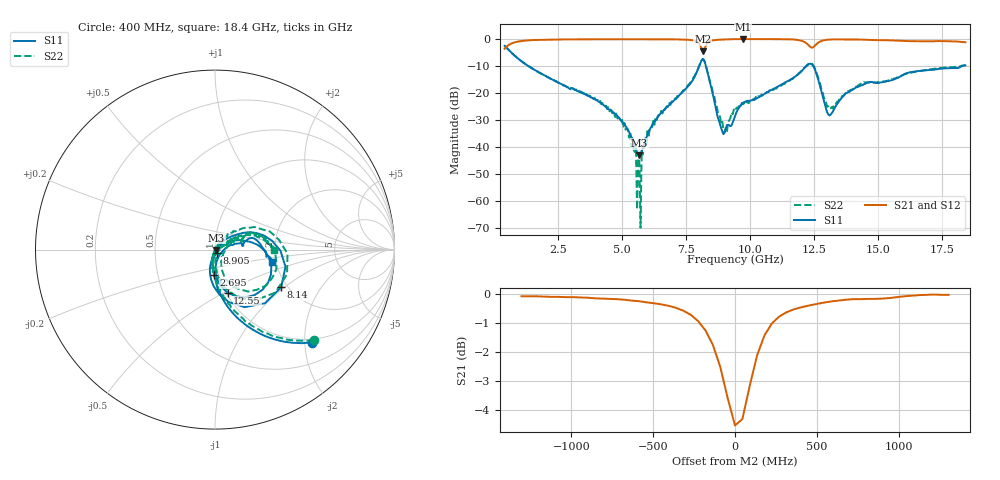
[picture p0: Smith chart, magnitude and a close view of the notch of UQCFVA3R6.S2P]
!  Part Number  UQCFVA3R6  Mounting Orientation: Horizontal
!  Description: Ultra Low ESR Microwave capacitors
!  Application: Coupling, Bypass, Tuning, DC Block
!  Filters, Matching
# GHZ S DB R 50
! Freq  |S11|  S11 Ph  |S21|  S21 Ph  |S12|  S12 Ph  |S22|  S22 Ph
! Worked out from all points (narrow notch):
!   401 points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, 400 MHz to 18.4 GHz, reference 50 ohm
!   highest |S21| = -0.01 dB at 9.715 GHz (marker M1); lowest = -4.5 dB at 8.14 GHz (marker M2)
!   notch at M2: 4.4 dB deep, 225 MHz wide at half that depth
!   lowest |S11| = -43.2 dB at 5.665 GHz (marker M3), VSWR 1.01, Z = 50.6 - j0.26 ohm
!   |S11| at or under -10 dB: 1.323 GHz to 8 GHz (6.676 GHz wide, 143 % of centre); 8.264 GHz to 12.2 GHz (3.932 GHz wide, 38.4 % of centre); 12.46 GHz to 18.29 GHz (5.837 GHz wide, 38 % of centre)
!   |S22| runs from -70.0 to -2.5 dB; largest |S21 - S12| = 0.0053
!   S11 on the Smith chart (normalised r, x): 400 MHz: 0.92, -2.15; 2.695 GHz: 0.95, -0.27; 8.14 GHz: 1.85, -0.95; 8.905 GHz: 1.02, -0.03; 12.55 GHz: 1.02, -0.52; 18.4 GHz: 1.89, -0.30
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0.4  -2.53 -43.9  -3.59 46.6  -3.60 46.6  -2.54 -42.6
1.12  -8.66 -74.2  -0.66 16.8  -0.67 16.8  -8.72 -71.6
2.695  -17.04 -91.6  -0.15 -3.1  -0.16 -3.1  -17.30 -90.5
3.415  -20.02 -96.5  -0.10 -9.1  -0.11 -9.0  -19.69 -95.4
5.08  -31.68 -94.4  -0.06 -19.7  -0.07 -19.6  -31.12 -106.3
5.44  -38.57 -77.2  -0.04 -21.9  -0.05 -21.9  -41.08 -74.8
5.665  -43.20 -21.8  -0.04 -23.3  -0.04 -23.3  -45.68 35.6
5.845  -39.20 24.0  -0.04 -24.5  -0.04 -24.5  -40.58 27.6
6.43  -28.40 45.5  -0.07 -28.4  -0.07 -28.3  -28.12 60.0
7.87  -13.01 25.6  -0.73 -44.4  -0.72 -44.2  -12.78 32.1
8.14  -7.44 -29.7  -4.55 -39.4  -4.55 -39.3  -7.45 -18.8
8.41  -15.55 -97.7  -0.79 -26.3  -0.77 -26.2  -15.39 -80.7
8.905  -34.40 -58.2  -0.19 -35.2  -0.17 -35.1  -30.76 -57.1
9.4  -28.58 31.0  -0.04 -39.4  -0.02 -39.4  -26.75 26.3
9.715  -23.69 26.1  -0.01 -41.7  -0.01 -41.7  -24.22 27.9
11.875  -13.01 8.7  -0.37 -61.2  -0.35 -61.2  -12.98 19.6
12.415  -9.48 -49.1  -3.20 -56.1  -3.19 -56.1  -9.16 -35.1
12.55  -12.04 -73.6  -2.19 -47.5  -2.19 -47.4  -11.67 -58.0
13.09  -28.37 -36.7  -0.20 -55.0  -0.19 -55.1  -25.96 -26.4
14.08  -18.24 15.8  -0.12 -64.7  -0.11 -64.8  -18.35 25.2
15.43  -15.54 14.0  -0.46 -73.6  -0.45 -73.7  -15.32 24.9
18.4  -9.81 -12.7  -1.19 -90.7  -1.17 -90.9  -9.71 -0.1
